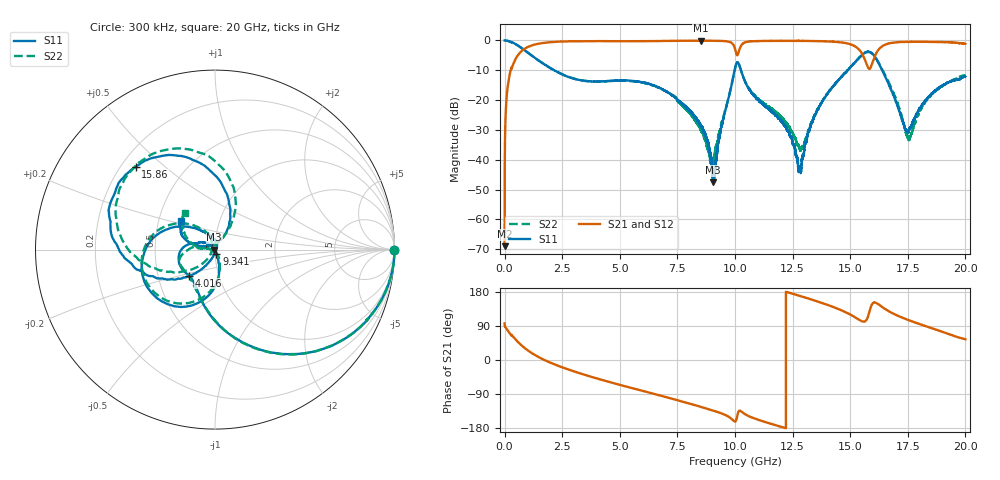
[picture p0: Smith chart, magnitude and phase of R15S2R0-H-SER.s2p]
!{R15S2R0}
!Johanson Technology Inc.
!www.johansontechnology.com
!Test Board Conditions:
!Substrate Type  RO4350B
!Substrate Thickness  20 mil
!Substrate Dk  3.66
!TL Type: GCPW
!TL Trace Width  34 mil
!TL Gap  10 mil
!Electrode orientation  Horizontal
!DUT TOPOLOGY	SERIES
!Mounting Pad LxW  26x52 mil
! Created Sat Feb  6 13:48:20 2021
# hz S ma R 50
! 2 Port Network Data from SP1.SP block
! freq  magS11  angS11  magS21  angS21  magS12  angS12  magS22  angS22
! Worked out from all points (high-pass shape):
!   20001 points, 300 kHz to 20 GHz, reference 50 ohm
!   highest |S21| = -0.08 dB at 8.504 GHz (marker M1); lowest = -69.0 dB at 300 kHz (marker M2)
!   |S21| within 3 dB of the highest: 815.9 MHz to 10.01 GHz (9.196 GHz wide, 170 % of centre); 10.19 GHz to 15.38 GHz (5.194 GHz wide, 40.6 % of centre)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
!   lowest |S11| = -47.5 dB at 9.053 GHz (marker M3), VSWR 1.01, Z = 49.6 - j0.0196 ohm
!   |S11| at or under -10 dB: 2.157 GHz to 9.981 GHz (7.824 GHz wide, 129 % of centre); 10.26 GHz to 14.89 GHz (4.628 GHz wide, 36.8 % of centre); 16.39 GHz to end of sweep
!   |S22| runs from -41.7 to 0.0 dB; largest |S21 - S12| = 0.014
!   S11 on the Smith chart (normalised r, x): 300 kHz: open; 4.016 GHz: 0.72, -0.22; 9.341 GHz: 1.01, -0.05; 15.86 GHz: 0.26, +0.40; 20 GHz: 0.65, +0.22
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300000  1 -0.3  0.0003565 96.5  0.0004209 90.1  0.998 -0.2
1.303e8  0.9857 -11.3  0.1634 78.4  0.1641 78.4  0.9854 -11.3
4.823e8  0.8666 -36.0  0.4938 53.7  0.4953 53.7  0.866 -36.1
1.5643e9  0.4374 -85.1  0.8937 4.9  0.8955 4.9  0.4379 -84.8
3.3343e9  0.2142 -124.3  0.973 -36.3  0.9725 -36.4  0.2152 -127.9
4.0163e9  0.2057 -135.4  0.975 -48.9  0.9747 -48.9  0.2051 -141.8
6.6673e9  0.1643 172.1  0.9777 -92.4  0.979 -92.4  0.1635 -176.5
8.5043e9  0.03725 137.6  0.9914 -123.4  0.989 -123.3  0.03269 173.6
9.0533e9  0.004211 -177.3  0.9878 -133.4  0.9871 -133.4  0.00881 -101.8
9.3413e9  0.02633 -73.5  0.9827 -139.2  0.9838 -139.3  0.03039 -63.6
1.00003e10  0.3432 -114.0  0.7268 -162.5  0.7274 -162.3  0.3365 -117.5
1.03703e10  0.2372 147.2  0.9042 -140.3  0.9039 -140.2  0.2376 141.5
1.22533e10  0.03138 72.4  0.9854 179.2  0.9839 179.3  0.04079 115.1
1.28013e10  0.007451 -17.3  0.983 169.3  0.9813 169.5  0.01554 160.9
1.33343e10  0.0418 -104.8  0.9787 159.3  0.98 159.4  0.04348 -130.6
1.50823e10  0.3764 -156.9  0.8438 117.2  0.8421 117.3  0.386 -167.0
1.58563e10  0.6403 133.7  0.3381 132.1  0.3378 131.9  0.6368 123.7
1.62143e10  0.4289 92.1  0.6877 147.5  0.6901 147.9  0.4368 82.3
1.66673e10  0.1867 63.1  0.8904 128.7  0.8864 129.4  0.2018 59.5
1.75373e10  0.02982 121.8  0.9496 105.4  0.9468 105.4  0.02239 115.4
1.84733e10  0.119 165.8  0.9475 85.3  0.9462 85.4  0.1172 168.7
2e10  0.2485 139.6  0.879 54.7  0.8737 54.6  0.2618 129.0
